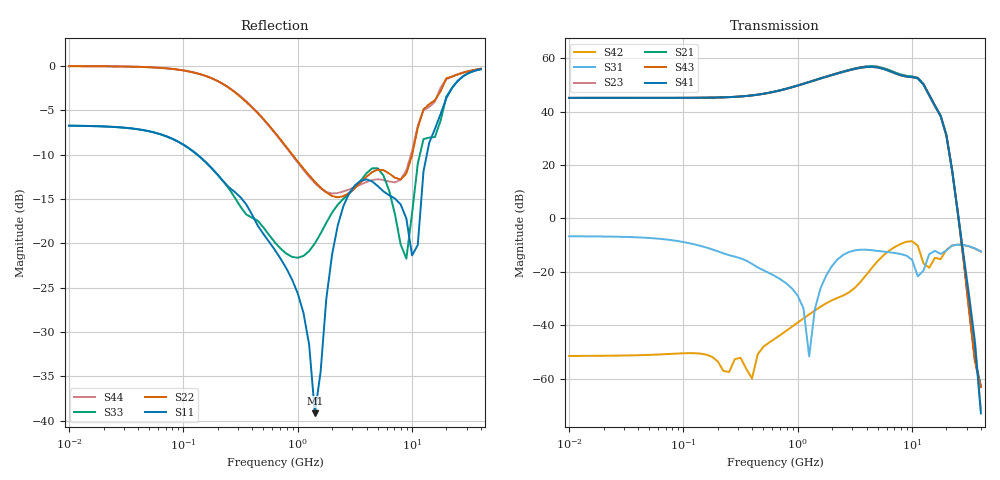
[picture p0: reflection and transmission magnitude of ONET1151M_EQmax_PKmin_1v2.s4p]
! Touchstone Ver. 1.0
! Thu Sep  6 15:40:26 2012
! Number of ports is 4
# Hz	S	DB	R	50.000000
! SCATTERING PARAMETERS  :
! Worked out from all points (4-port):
!   73 points, 10 MHz to 40 GHz, reference 50 ohm
!   strongest paths, dB at 10 MHz, 79.43 MHz, 631 MHz, 5.012 GHz, 40 GHz:
!     S41: 45.1, 45.2, 47.5, 56.5, -73.0
!     S43: 45.1, 45.2, 47.5, 56.5, -63.1
!     S21: 45.2, 45.2, 47.5, 56.8, -62.8
!     S23: 45.2, 45.2, 47.5, 56.8, -71.6
!     S31: -6.7, -8.1, -21.6, -12.2, -12.4
!     S42: -51.5, -50.7, -45.0, -15.9, -12.4
!   lowest |S11| = -39.1 dB at 1.413 GHz (marker M1), VSWR 1.02, Z = 49.1 - j0.607 ohm
!   |S11| at or under -10 dB: 132.2 MHz to 13.49 GHz (13.36 GHz wide, 196 % of centre)
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1e7  -6.75 -4.6  -110.77 178.2  -6.68 -4.3  -110.73 178.2
     45.16 -175.3  -0.04 7.1  45.16 4.7  -51.60 9.7
     -6.67 -4.3  -110.75 178.1  -6.75 -4.6  -110.75 178.3
     45.14 4.7  -51.49 9.9  45.14 -175.3  -0.04 7.1
1.412538e9  -39.15 -145.9  -42.47 74.9  -21.68 -51.3  -42.40 74.9
            51.83 159.5  -13.06 -83.0  51.83 -20.5  -38.40 58.3
            -33.85 86.6  -42.43 75.0  -20.01 -65.6  -42.40 75.0
            51.74 -21.2  -34.45 51.9  51.73 158.7  -13.22 -81.4
3.162278e9  -13.46 -49.0  -38.06 1.8  -15.64 129.3  -38.01 2.0
            56.17 71.8  -13.77 -98.8  56.16 -108.2  -25.14 -62.8
            -11.95 -37.1  -38.04 2.1  -13.76 144.5  -38.00 1.8
            56.00 -109.3  -25.96 -78.6  55.99 70.7  -13.67 -102.8
4.466836e9  -13.01 -144.3  -38.38 -14.5  -12.46 32.7  -38.33 -14.2
            57.03 0.8  -11.98 -131.7  57.02 -179.2  -16.94 -141.9
            -11.90 -131.3  -38.35 -14.1  -11.55 45.3  -38.32 -14.4
            56.77 179.6  -18.41 -149.2  56.75 -0.4  -12.87 -134.1
7.943282e9  -15.61 14.0  -38.35 -61.1  -18.51 148.1  -38.30 -60.7
            53.91 -166.1  -12.80 145.2  53.90 14.0  -8.84 93.9
            -13.32 56.2  -38.36 -60.5  -20.11 -128.7  -38.25 -61.1
            53.63 13.5  -9.55 96.2  53.61 -166.4  -12.83 151.6
1.122018e10  -20.19 36.0  -40.11 -97.4  -15.47 35.6  -40.15 -96.3
             52.70 38.4  -7.00 86.5  52.68 -141.4  -10.37 11.4
             -21.66 -57.2  -40.19 -95.6  -11.03 53.2  -40.06 -97.9
             52.45 -142.2  -10.18 14.0  52.43 38.0  -6.76 84.6
4e10  -0.38 -143.6  -68.86 138.2  -12.36 -53.0  -68.66 138.1
      -62.81 -172.9  -0.33 -143.9  -71.64 -75.3  -12.41 -53.2
      -12.36 -53.0  -68.58 137.8  -0.38 -143.6  -68.84 138.4
      -72.99 -82.9  -12.40 -53.3  -63.15 -171.6  -0.33 -143.9
